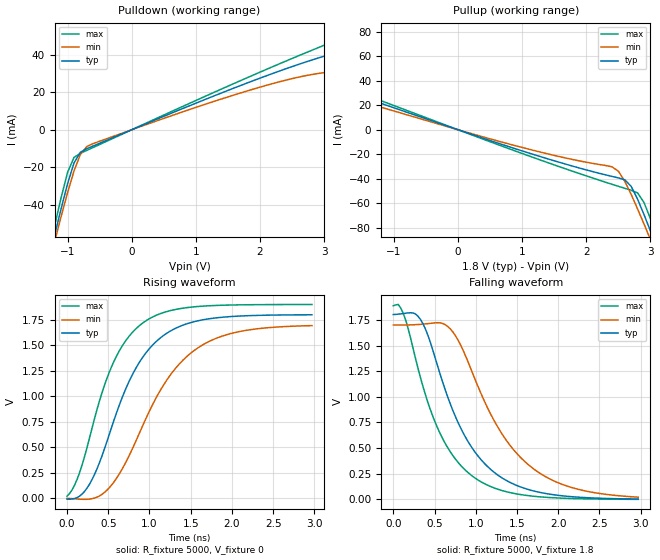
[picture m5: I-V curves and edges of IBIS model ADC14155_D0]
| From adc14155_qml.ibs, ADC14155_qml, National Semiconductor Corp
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|   Driver Outputs Model ADC14155_D0
[Model]   ADC14155_D0
Model_type Output
Polarity Non-Inverting
Vmeas=0.9
|Cref=5p
Rref=50
C_comp   1.891p   1.832p   1.953p
|   TYP   MIN   MAX
[Temperature Range]   25   85   -40
[Pullup Reference]   1.8   1.7   1.9
[Pulldown Reference]   0   0   0
[POWER clamp Reference]   3.3   3.0   3.6
[GND clamp Reference]   0   0   0
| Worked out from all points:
|   slope of the pulldown table from 0 to 0.27 V, typ, clamps not added: 69.7 ohm
|   slope of the pullup table from 0 to 0.27 V, typ, clamps not added: 56.5 ohm
|   falling waveform, R_fixture 5000, V_fixture 1.8: 20-80 % time 607ps typ, 716ps min, 540ps max; typ from 1.8 V to 0.004 V
|   rising waveform, R_fixture 5000, V_fixture 0: 20-80 % time 574ps typ, 703ps min, 486ps max; typ from -0.01 V to 1.8 V
[Pullup]
|V(PullUp)   I(typ)   I(min)   I(max)
-4.8V     441.5mA    449.8mA    410.3mA
-2.9V     121.1mA    146.1mA    90.84mA
-2.7V     89.19mA    115.4mA    60.05mA
-2.5V     59.37mA    85.45mA    49.41mA
-2.3V     41.81mA    57.06mA    45.38mA
-2V       35.93mA    31.14mA    39.4mA
2.4V      -38.03mA   -30.2mA    -44.45mA
2.7V      -46.14mA   -52.78mA   -49.32mA
2.8V      -56.66mA   -64.59mA   -51.48mA
3V        -82.49mA   -89.41mA   -72.48mA
3.1V      -96.09mA   -102.1mA   -87.06mA
5V        -367.8mA   -362.9mA   -377.2mA
[Pulldown]
|V(pulldown)   I(typ)   I(min)   I(max)
-3.3V     -374.3mA   -358.5mA   -391mA
-1.3V     -70.14mA   -72.65mA   -66.11mA
-1.2V     -55.76mA   -59.17mA   -50.73mA
-1V       -28.64mA   -33.41mA   -22.64mA
-900mV    -17.64mA   -21.89mA   -14.71mA
-700mV    -10.05mA   -8.912mA   -10.97mA
2.1V      28.71mA    23.63mA    32.11mA
3.7V      44.18mA    33.18mA    53.97mA
3.8V      44.6mA     36.5mA     55.12mA
4V        45.35mA    57.44mA    57.2mA
4.3V      61.8mA     99.94mA    59.56mA
6.5V      424.3mA    449.7mA    392.1mA
|VT Tables are generated with Cref=5pF
[Ramp]
dV/dt_r   1.084/579.34p   1.020/712.54p   1.143/492.70p
dV/dt_f   1.084/612.14p   1.020/740.37p   1.143/544.06p
R_load=50
[Falling Waveform]
R_fixture=5000
V_fixture=1.8
V_fixture_min=1.7
V_fixture_max=1.9
| time   V (typ)   V(min)   V(max)
0s        1.802V     1.7V       1.888V
120ps     1.812V     1.7V       1.816V
330ps     1.754V     1.707V     1.187V
480ps     1.454V     1.719V     809.1mV
660ps     999.3mV    1.686V     504.4mV
930ps     534mV      1.294V     246mV
1.29ns    224.9mV    675.2mV    93.73mV
1.68ns    87.23mV    311.2mV    32.92mV
2.19ns    25.19mV    110.1mV    8.375mV
2.97ns    3.753mV    22.19mV    1.03mV
[Rising Waveform]
R_fixture= 5000
V_fixture= 0
V_fixture_min= 0
V_fixture_max= 0
| time   V (typ)   V(min)   V(max)
0s        -10.29mV   -2.48mV    19.11mV
120ps     4.498mV    -8.097mV   179.9mV
240ps     95.3mV     -11.37mV   488.5mV
480ps     545.4mV    74.71mV    1.167V
660ps     968.5mV    273.3mV    1.481V
900ps     1.361V     678.2mV    1.707V
1.23ns    1.628V     1.182V     1.835V
1.62ns    1.745V     1.491V     1.882V
2.13ns    1.788V     1.64V      1.897V
2.97ns    1.799V     1.692V     1.9V
